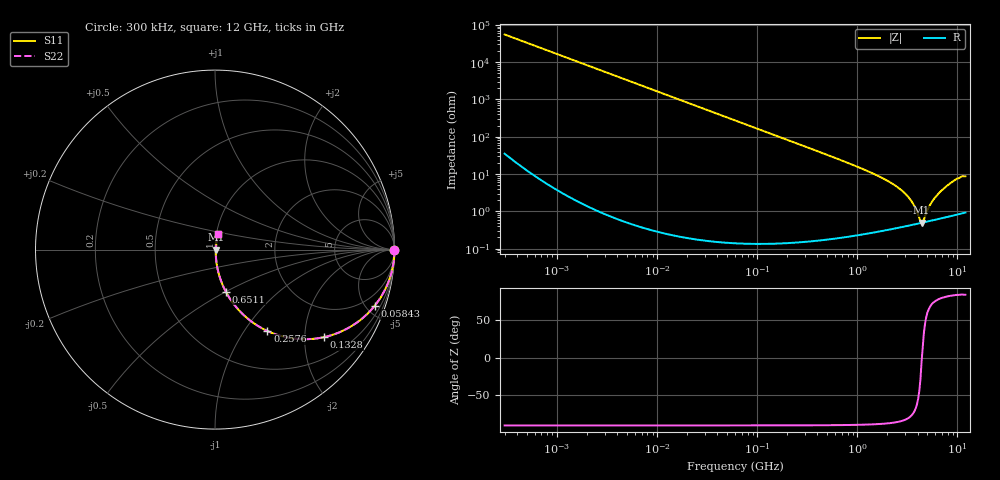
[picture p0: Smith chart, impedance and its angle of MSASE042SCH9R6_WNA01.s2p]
! MSASE042SCH9R6_WNA01  S-PARAMETER MODEL  ( General Type )
! Model Generated by TAIYO YUDEN Corporation (http://www.ty-top.com)
! Version 1.0
! TAIYO YUDEN Control No. 120810
! Copyright(c) 2012 TAIYO YUDEN CO.,LTD. All Rights Reserved.
! Product Description (link to TY-COMPAS)
! https://ds.yuden.co.jp/TYCOMPAS/or/detail?pn=MSASE042SCH9R6BWNA01&u=M
! Products Name : Multilayer Ceramic Capacitors
! Characteristics :
!  Capacitance : 9.6 pF , Rated Voltage : 16V , TCC : CH / C0H
!  Case Size : 0.4 x 0.2 / 0.016 x 0.008 [mm/inch] , Thickness : 0.2 / 0.008 [mm/inch]
!  (Conditions: Temperature = 25 degC , DC Bias Current/Voltage = 0A / 0V)
! External Node Assignments :
!  1  o---| |---o  2
! GND o---------o GND
! Frequency Range : 0.3MHz  -  12000MHz  [ 401 STEP ]
# MHz S RI R 50
! Freq[MHz].  S11 Real  S11 Imag  S21 Real  S21 Imag  S12 Real  S12 Imag  S22 Real  S22 Imag
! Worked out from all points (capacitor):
!   401 points, 300 kHz to 12 GHz, reference 50 ohm
!   read as one part in series: C = 9.6 pF near 316.3 kHz
!   lowest |Z| = 494 mohm at 4.385 GHz (marker M1)
!   series resonance near 4.411 GHz, so ESL is about 140 pH
!   S11 on the Smith chart (normalised r, x): 300 kHz: open; 58.43 MHz: 1.00, -5.68; 132.8 MHz: 1.00, -2.49; 257.6 MHz: 1.00, -1.28; 651.1 MHz: 1.00, -0.50; 12 GHz: 1.02, +0.17
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0.3  1 -0.00181  4.42e-06 0.00181  4.42e-06 0.00181  1 -0.00181
1.769972  0.9999 -0.0107  0.000116 0.0107  0.000116 0.0107  0.9999 -0.0107
10.44266  0.996 -0.0627  0.00396 0.0627  0.00396 0.0627  0.996 -0.0627
25.70316  0.9765 -0.1513  0.0235 0.1513  0.0235 0.1513  0.9765 -0.1513
58.43137  0.8894 -0.3134  0.1106 0.3134  0.1106 0.3134  0.8894 -0.3134
60  0.8841 -0.3198  0.1159 0.3198  0.1159 0.3198  0.8841 -0.3198
132.8329  0.6087 -0.4875  0.3913 0.4875  0.3913 0.4875  0.6087 -0.4875
257.5933  0.2921 -0.4536  0.7079 0.4536  0.7079 0.4536  0.2921 -0.4536
353.9943  0.1789 -0.3816  0.8211 0.3816  0.8211 0.3816  0.1789 -0.3816
651.0506  0.0601 -0.2338  0.9399 0.2338  0.9399 0.2338  0.0601 -0.2338
1296.429  0.0159 -0.1148  0.9841 0.1148  0.9841 0.1148  0.0159 -0.1148
2088.533  0.00699 -0.0611  0.993 0.0611  0.993 0.0611  0.00699 -0.0611
2650.866  0.00526 -0.0397  0.9947 0.0397  0.9947 0.0397  0.00526 -0.0397
3190.978  0.00469 -0.0247  0.9953 0.0247  0.9953 0.0247  0.00469 -0.0247
3642.919  0.00461 -0.0145  0.9954 0.0145  0.9954 0.0145  0.00461 -0.0145
4158.869  0.00477 -0.00455  0.9952 0.00455  0.9952 0.00455  0.00477 -0.00455
4385.161  0.00491 -0.000379  0.9951 0.000379  0.9951 0.000379  0.00491 -0.000379
4623.766  0.00507 0.00337  0.9949 -0.00337  0.9949 -0.00337  0.00507 0.00337
5565.855  0.00595 0.017  0.994 -0.017  0.994 -0.017  0.00595 0.017
6699.894  0.00739 0.0322  0.9926 -0.0322  0.9926 -0.0322  0.00739 0.0322
9454.42  0.0126 0.0679  0.9874 -0.0679  0.9874 -0.0679  0.0126 0.0679
12000  0.0165 0.0845  0.9835 -0.0845  0.9835 -0.0845  0.0165 0.0845
